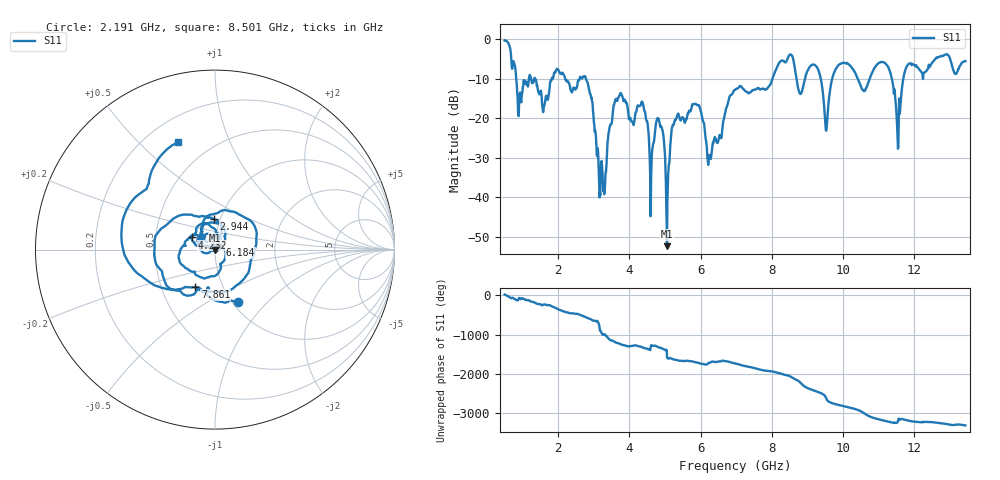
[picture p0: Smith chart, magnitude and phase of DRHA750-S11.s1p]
# Hz S DB R 50
! HP 8720B Vector Network Analyzer
! S-Parameter: S11
! Start Frequency: 490 MHz
! Stop Frequency: 13450 MHz
! Number of Points: 1601
! Date: 26-Mar-2022 11:25:31
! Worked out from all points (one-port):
!   1601 points, 490 MHz to 13.45 GHz, reference 50 ohm
!   lowest |S11| = -52.3 dB at 5.058 GHz (marker M1), VSWR 1.00, Z = 49.8 - j0.168 ohm
!   |S11| at or under -10 dB: 1.34 GHz to 1.817 GHz (476.7 MHz wide, 30.2 % of centre); 2.195 GHz to 2.598 GHz (402.9 MHz wide, 16.8 % of centre); 2.779 GHz to 8.02 GHz (5.242 GHz wide, 97.1 % of centre)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
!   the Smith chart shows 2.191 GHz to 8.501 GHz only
!   S11 on the Smith chart (normalised r, x): 2.191 GHz: 1.06, -0.69; 2.944 GHz: 0.93, +0.33; 4.232 GHz: 0.77, +0.11; 6.184 GHz: 1.06, +0.05; 7.861 GHz: 0.74, -0.33; 8.501 GHz: 0.33, +0.66
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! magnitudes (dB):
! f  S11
! 490 MHz  -0.3
! 911.2 MHz  -13.9
! 2.11 GHz  -8.5
! 2.191 GHz  -9.9
! 2.944 GHz  -15.3
! 3.228 GHz  -31.8
! 3.73 GHz  -14.1
! 4.232 GHz  -16.7
! 4.621 GHz  -31.5
! 4.872 GHz  -22.2
! 5.058 GHz  -52.3
! 5.35 GHz  -19.2
! 5.925 GHz  -16.7
! 6.184 GHz  -28.4
! 6.97 GHz  -12.8
! 7.861 GHz  -12.6
! 8.501 GHz  -4.0
! 8.59 GHz  -4.5
! 8.809 GHz  -13.8
! 9.278 GHz  -7.1
! 9.538 GHz  -23.1
! 9.789 GHz  -7.8
! 10.21 GHz  -6.7
! 10.6 GHz  -13.1
! 11.22 GHz  -6.3
! 11.56 GHz  -27.0
! 11.83 GHz  -6.4
! 13.45 GHz  -5.5
